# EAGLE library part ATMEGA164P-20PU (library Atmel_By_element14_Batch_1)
8-bit Microcontroller with 16K/32K/64K Bytes In-System Programmable Flash
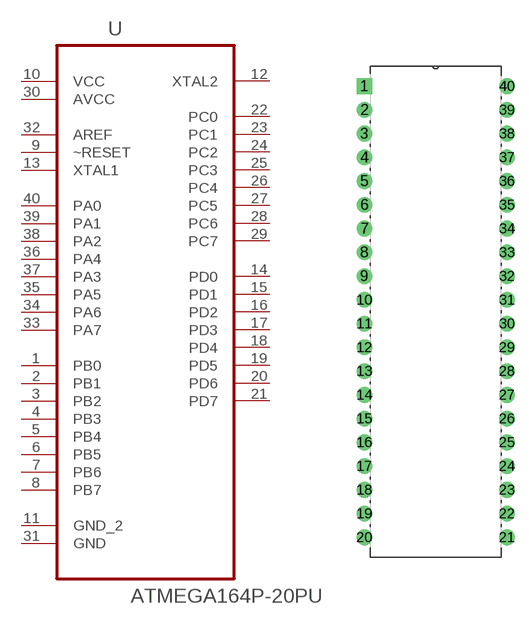
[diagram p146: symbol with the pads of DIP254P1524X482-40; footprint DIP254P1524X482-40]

Designator prefix U

## ATMEGA164P-20PU (MPN: ATMEGA164P-20PU; OC_FARNELL: 1455099; OC_NEWARK: 58M3726; PACKAGE: DIP-40; SUPPLIER: Atmel)  [DIP254P1524X482-40]
1  PB0
2  PB1
3  PB2
4  PB3
5  PB4
6  PB5
7  PB6
8  PB7
9  ~RESET  in
10  VCC  pwr
11  GND_2  pas
12  XTAL2  out
13  XTAL1  in
14  PD0
15  PD1
16  PD2
17  PD3
18  PD4
19  PD5
20  PD6
21  PD7
22  PC0
23  PC1
24  PC2
25  PC3
26  PC4
27  PC5
28  PC6
29  PC7
30  AVCC  pwr
31  GND  pas
32  AREF  in
33  PA7
34  PA6
35  PA5
36  PA4
37  PA3
38  PA2
39  PA1
40  PA0

## Footprint DIP254P1524X482-40 (pad centres in mm)
drill 1.118 square: 1 -15.24,48.26
drill 1.118: 2 -15.24,45.72; 3 -15.24,43.18; 4 -15.24,40.64; 5 -15.24,38.1; 6 -15.24,35.56; 7 -15.24,33.02; 8 -15.24,30.48; 9 -15.24,27.94; 10 -15.24,25.4; 11 -15.24,22.86; 12 -15.24,20.32; 13 -15.24,17.78; 14 -15.24,15.24; 15 -15.24,12.7; 16 -15.24,10.16; 17 -15.24,7.62; 18 -15.24,5.08; 19 -15.24,2.54; 20 -15.24,0; 21 0,0; 22 0,2.54; 23 0,5.08; 24 0,7.62; 25 0,10.16; 26 0,12.7; 27 0,15.24; 28 0,17.78; 29 0,20.32; 30 0,22.86; 31 0,25.4; 32 0,27.94; 33 0,30.48; 34 0,33.02; 35 0,35.56; 36 0,38.1; 37 0,40.64; 38 0,43.18; 39 0,45.72; 40 0,48.26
